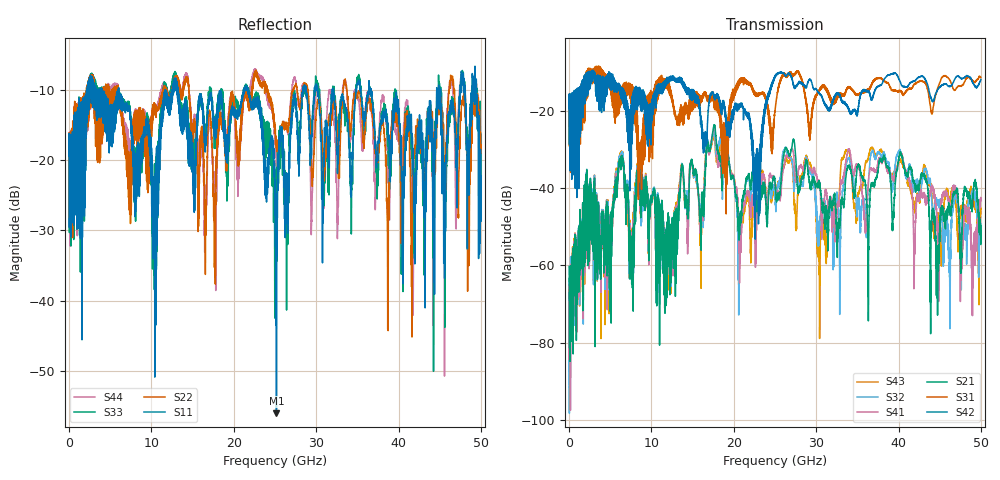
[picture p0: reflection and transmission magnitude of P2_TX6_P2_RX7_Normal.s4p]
!Keysight Technologies,N5225B,MY57041031,A.13.20.10
!Date: Friday, May 31, 2019 11:38:03
!Correction: S11(Full 4 Port(1,2,3,4))
!S12(Full 4 Port(1,2,3,4))
!S13(Full 4 Port(1,2,3,4))
!S14(Full 4 Port(1,2,3,4))
!S21(Full 4 Port(1,2,3,4))
!S22(Full 4 Port(1,2,3,4))
!S23(Full 4 Port(1,2,3,4))
!S24(Full 4 Port(1,2,3,4))
!S31(Full 4 Port(1,2,3,4))
!S32(Full 4 Port(1,2,3,4))
!S33(Full 4 Port(1,2,3,4))
!S34(Full 4 Port(1,2,3,4))
!S41(Full 4 Port(1,2,3,4))
!S42(Full 4 Port(1,2,3,4))
!S43(Full 4 Port(1,2,3,4))
!S44(Full 4 Port(1,2,3,4))
!S4P File: Measurements: <S11,S12,S13,S14>,
!<S21,S22,S23,S24>,
!<S31,S32,S33,S34>,
!<S41,S42,S43,S44>:
# Hz S  dB  R 50.0
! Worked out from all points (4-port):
!   5000 points, 10 MHz to 50 GHz, reference 50 ohm
!   strongest paths, dB at 10 MHz, 12.51 GHz, 25.01 GHz, 37.51 GHz, 50 GHz:
!     S42: -19.4, -12.1, -11.4, -13.8, -12.0
!     S31: -19.4, -16.8, -20.0, -11.7, -11.5
!     S21: -60.2, -55.2, -38.9, -35.5, -49.7
!     S41: -65.1, -59.6, -39.0, -33.3, -42.5
!     S32: -65.2, -58.1, -42.8, -30.8, -50.4
!     S43: -73.8, -59.4, -42.8, -31.0, -45.2
!   lowest |S11| = -56.0 dB at 25.18 GHz (marker M1), VSWR 1.00, Z = 50 - j0.154 ohm
!   |S11| at or under -10 dB: 13.21 GHz to 21.26 GHz (8.054 GHz wide, 46.7 % of centre); 21.73 GHz to 28.41 GHz (6.676 GHz wide, 26.6 % of centre); 36.66 GHz to 44.63 GHz (7.968 GHz wide, 19.6 % of centre)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
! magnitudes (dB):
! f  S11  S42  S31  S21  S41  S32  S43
! 10 MHz  -19.4  -19.4  -19.4  -60.2  -65.1  -65.2  -73.8
! 6.32 GHz  -11.1  -14.0  -14.0  -34.2  -33.5  -32.5  -31.8
! 7.59 GHz  -16.4  -18.7  -17.1  -54.9  -52.5  -55.7  -52.5
! 17.55 GHz  -14.8  -16.1  -16.5  -24.1  -24.5  -25.4  -26.3
! 22.8 GHz  -12.1  -36.9  -15.6  -43.6  -46.8  -41.4  -44.4
! 25.18 GHz  -56.0  -10.5  -16.9  -43.1  -41.0  -43.2  -40.6
! 50 GHz  -22.2  -12.0  -11.5  -49.7  -42.5  -50.4  -45.2
